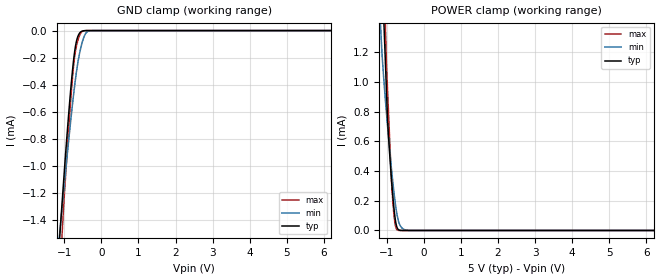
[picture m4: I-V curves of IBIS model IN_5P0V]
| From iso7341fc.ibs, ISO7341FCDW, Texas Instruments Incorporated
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|   IN_5P0V Model
[Model]   IN_5P0V
Model_type   Input
Vinl = 0.8
Vinh = 2
|   typ   min   max
|   (nom PVT)   (slow PVT)   (fast PVT)
C_comp   0.354pF   0.325pF   0.383pF
| Where   nom PVT is  Nominal Process, 5.0V, 27C
|   Fast PVT is Strong Process, 5.5V, -40C
|   Slow PVT is Weak Process, 4.5V, 150C
[Voltage Range]   5   4.5   5.5
[Temperature Range]   27   150   -40
[Power Clamp Reference]   5   4.5   5.5
[GND Clamp Reference]   0   0   0
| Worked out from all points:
|   GND clamp passes 1 mA (typ) near -0.99 V on its own axis
|   POWER clamp passes 1 mA (typ) near -1.02 V on its own axis
[GND Clamp]
|   Voltage   I(typ)   I(min)   I(max)
-5V       -17.38mA   -13.33mA   -21.61mA
-1.115V   -1.488mA   -1.468mA   -1.779mA
-1.055V   -1.255mA   -1.295mA   -1.484mA
-1.01V    -1.081mA   -1.167mA   -1.262mA
-875mV    -592.5uA   -792.6uA   -699.4uA
-755mV    -232uA     -485.3uA   -275uA
-710mV    -135.1uA   -382.4uA   -171.3uA
-650mV    -56.09uA   -263.4uA   -88.85uA
-515mV    -3.659uA   -84.59uA   -6.851uA
-410mV    -199.6nA   -16.03uA   -230.9nA
-290mV    0A         -798.1nA   0A
10V       0A         0A         0A
[POWER Clamp]
|   Voltage   I(typ)   I(min)   I(max)
-5V       33.77mA    25.3mA     41.21mA
-1.34V    3.142mA    2.182mA    4.333mA
-1.13V    1.742mA    1.192mA    2.29mA
-1.07V    1.343mA    978.4uA    1.706mA
-1.04V    1.143mA    881.8uA    1.414mA
-980mV    743.1uA    701.8uA    947uA
-875mV    346.2uA    416.8uA    332.1uA
-785mV    98.85uA    210uA      56.71uA
-710mV    12.46uA    88.64uA    2.617uA
-605mV    271.7nA    20.55uA    16.4nA
-425mV    0A         597.4nA    0A
10V       0A         0A         0A
